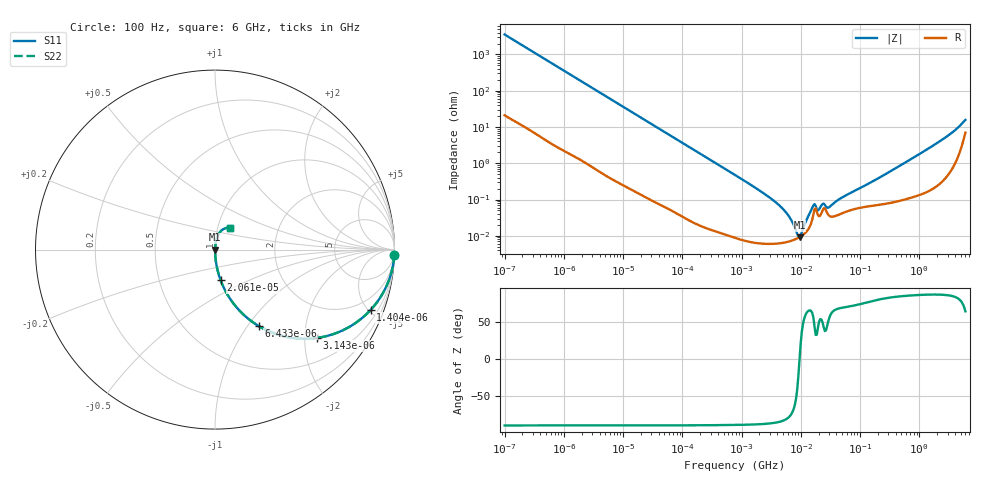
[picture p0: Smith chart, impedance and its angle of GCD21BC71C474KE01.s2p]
!Murata Part Number: GCD21BC71C474KE01
!These Parameters are Measured in Series Mode Connection
!Data Generated on Mar 13, 2026
!  o--ll--o
!Port1  Port2
!  o------o
!Operation Temp=25[degC], DC Bias Voltage=0[V]
!Freq. Start=100[Hz] Stop=6[GHz] 401[Steps]
# Hz S RI R 50
!Freq.(Hz) S11(Real) S11(Imag) S21(Real) S21(Imag) S12(Real) S12(Imag) S22(Real) S22(Imag)
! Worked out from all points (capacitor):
!   401 points, 100 Hz to 6 GHz, reference 50 ohm
!   read as one part in series: C = 446 nF near 109 Hz
!   lowest |Z| = 9.16 mohm at 9.506 MHz (marker M1)
!   series resonance near 9.523 MHz, so ESL is about 630 pH
!   S11 on the Smith chart (normalised r, x): 100 Hz: 1, -71; 1.404 kHz: 1.03, -5.13; 3.143 kHz: 1.01, -2.30; 6.433 kHz: 1.01, -1.13; 20.61 kHz: 1.00, -0.35; 6 GHz: 1.14, +0.28
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100  0.999 -0.028  0.00095 0.028  0.00095 0.028  0.999 -0.028
438  0.9846 -0.1202  0.0154 0.1202  0.0154 0.1202  0.9846 -0.1202
1404  0.8666 -0.3368  0.1334 0.3368  0.1334 0.3368  0.8666 -0.3368
2008  0.762 -0.4226  0.238 0.4226  0.238 0.4226  0.762 -0.4226
3143  0.5692 -0.492  0.4308 0.492  0.4308 0.492  0.5692 -0.492
6433  0.2424 -0.4253  0.7576 0.4253  0.7576 0.4253  0.2424 -0.4253
20606  0.0315 -0.171  0.9685 0.171  0.9685 0.171  0.0315 -0.171
40335  0.00887 -0.0897  0.9911 0.0897  0.9911 0.0897  0.00887 -0.0897
774597  0.00011 -0.00476  0.9999 0.00476  0.9999 0.00476  0.00011 -0.00476
4440638  6.26e-05 -0.000663  0.9999 0.000663  0.9999 0.000663  6.26e-05 -0.000663
6353432  6.99e-05 -0.000332  0.9999 0.000332  0.9999 0.000332  6.99e-05 -0.000332
8692127  8.47e-05 -7.44e-05  0.9999 7.44e-05  0.9999 7.44e-05  8.47e-05 -7.44e-05
9506416  9.16e-05 -1.4e-06  0.9999 1.4e-06  0.9999 1.4e-06  9.16e-05 -1.4e-06
1.039699e7  0.000101 7.35e-05  0.9999 -7.35e-05  0.9999 -7.35e-05  0.000101 7.35e-05
1.555665e7  0.000277 0.000516  0.9997 -0.000516  0.9997 -0.000516  0.000277 0.000516
2.035112e7  0.000347 0.000412  0.9997 -0.000412  0.9997 -0.000412  0.000347 0.000412
2.434276e7  0.000571 0.000519  0.9994 -0.000519  0.9994 -0.000519  0.000571 0.000519
3.045065e7  0.000353 0.000516  0.9996 -0.000516  0.9996 -0.000516  0.000353 0.000516
5.211241e7  0.000432 0.00111  0.9996 -0.00111  0.9996 -0.00111  0.000432 0.00111
3.124326e8  0.000828 0.00573  0.9992 -0.00573  0.9992 -0.00573  0.000828 0.00573
2.34314e9  0.00475 0.0425  0.9953 -0.0425  0.9953 -0.0425  0.00475 0.0425
6e9  0.081 0.1212  0.919 -0.1212  0.919 -0.1212  0.081 0.1212
